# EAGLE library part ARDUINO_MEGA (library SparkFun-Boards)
Arduino Mega R3 ATmega2560 R3 compatible footprint. SparkFun Products: Arduino Mega 2560 R3
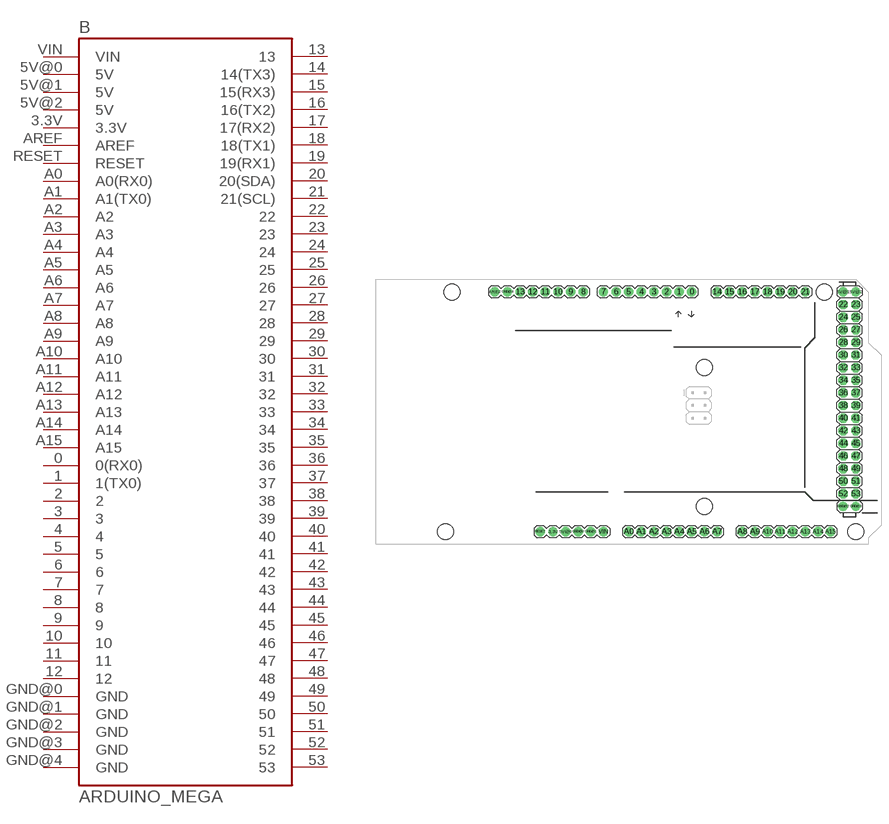
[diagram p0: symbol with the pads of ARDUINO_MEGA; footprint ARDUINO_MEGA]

Designator prefix B

## ARDUINO_MEGAFULL  [ARDUINO_MEGA]
0  0(RX0)
1  1(TX0)
2  2
3  3
3.3V  3.3V
4  4
5  5
5V@0  5V
5V@1  5V
5V@2  5V
6  6
7  7
8  8
9  9
10  10
11  11
12  12
13  13
14  14(TX3)
15  15(RX3)
16  16(TX2)
17  17(RX2)
18  18(TX1)
19  19(RX1)
20  20(SDA)
21  21(SCL)
22  22
23  23
24  24
25  25
26  26
27  27
28  28
29  29
30  30
31  31
32  32
33  33
34  34
35  35
36  36
37  37
38  38
39  39
40  40
41  41
42  42
43  43
44  44
45  45
46  46
47  47
48  48
49  49
50  50
51  51
52  52
53  53
A0  A0(RX0)
A1  A1(TX0)
A2  A2
A3  A3
A4  A4
A5  A5
A6  A6
A7  A7
A8  A8
A9  A9
A10  A10
A11  A11
A12  A12
A13  A13
A14  A14
A15  A15
AREF  AREF
GND@0  GND
GND@1  GND
GND@2  GND
GND@3  GND
GND@4  GND
RESET  RESET
VIN  VIN

## Footprint ARDUINO_MEGA (pad centres in mm)
Full Arduino MEGA footprint
drill 1.016 pad 1.88: 0 63.5,50.8; 1 60.96,50.8; 2 58.42,50.8; 3 55.88,50.8; 3.3V 35.56,2.54; 4 53.34,50.8; 5 50.8,50.8; 5V@0 38.1,2.54; 5V@1 93.98,50.8; 5V@2 96.52,50.8; 6 48.26,50.8; 7 45.72,50.8; 8 41.656,50.8; 9 39.116,50.8; 10 36.576,50.8; 11 34.036,50.8; 12 31.496,50.8; 13 28.956,50.8; 14 68.58,50.8; 15 71.12,50.8; 16 73.66,50.8; 17 76.2,50.8; 18 78.74,50.8; 19 81.28,50.8; 20 83.82,50.8; 21 86.36,50.8; A0 50.8,2.54; A1 53.34,2.54; A2 55.88,2.54; A3 58.42,2.54; A4 60.96,2.54; A5 63.5,2.54; A6 66.04,2.54; A7 68.58,2.54; A8 73.66,2.54; A9 76.2,2.54; A10 78.74,2.54; A11 81.28,2.54; A12 83.82,2.54; A13 86.36,2.54; A14 88.9,2.54; A15 91.44,2.54; AREF 23.876,50.8; GND@0 40.64,2.54; GND@1 43.18,2.54; GND@2 93.98,7.62; GND@3 96.52,7.62; GND@4 26.416,50.8; RESET 33.02,2.54; VIN 45.72,2.54
drill 1.016 pad 1.88 octagon: 22 93.98,48.26; 23 96.52,48.26; 24 93.98,45.72; 25 96.52,45.72; 26 93.98,43.18; 27 96.52,43.18; 28 93.98,40.64; 29 96.52,40.64; 30 93.98,38.1; 31 96.52,38.1; 32 93.98,35.56; 33 96.52,35.56; 34 93.98,33.02; 35 96.52,33.02; 36 93.98,30.48; 37 96.52,30.48; 38 93.98,27.94; 39 96.52,27.94; 40 93.98,25.4; 41 96.52,25.4; 42 93.98,22.86; 43 96.52,22.86; 44 93.98,20.32; 45 96.52,20.32; 46 93.98,17.78; 47 96.52,17.78; 48 93.98,15.24; 49 96.52,15.24; 50 93.98,12.7; 51 96.52,12.7; 52 93.98,10.16; 53 96.52,10.16
hole 3.2 at 15.24,50.8
hole 3.2 at 13.97,2.54
hole 3.2 at 66.04,35.56
hole 3.2 at 66.04,7.62
hole 3.2 at 90.17,50.8
hole 3.2 at 96.52,2.54

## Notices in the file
Licensing: Creative Commons ShareAlike 4.0 International - https://creativecommons.org/licenses/by-sa/4.0
